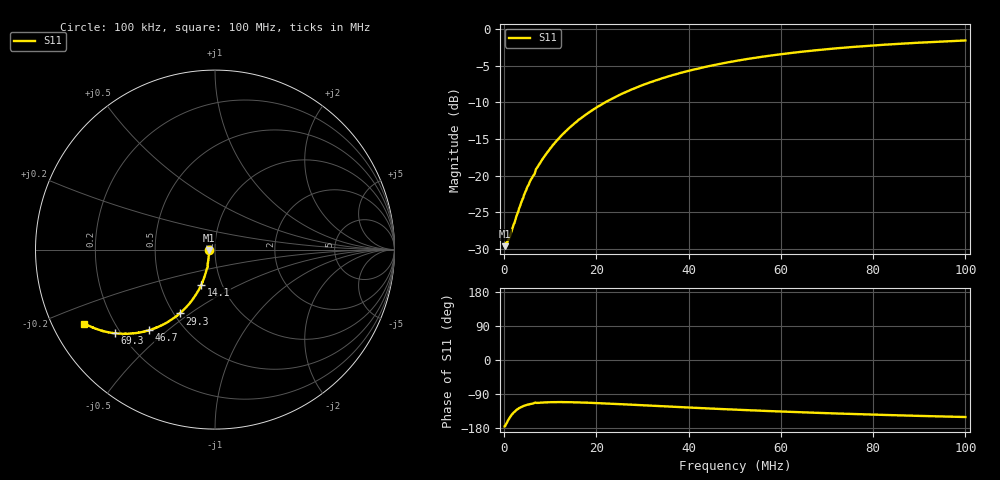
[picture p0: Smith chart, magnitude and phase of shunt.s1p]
# Hz S RI R 50.0
! written by SimSmith version 18.3h
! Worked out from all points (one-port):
!   1000 points, 100 kHz to 100 MHz, reference 50 ohm
!   lowest |S11| = -29.6 dB at 100 kHz (marker M1), VSWR 1.07, Z = 46.8 - j0.253 ohm
!   |S11| at or under -10 dB: start of sweep to 21.87 MHz
!   S11 on the Smith chart (normalised r, x): 100 kHz: 0.94, -0.01; 14.1 MHz: 0.80, -0.33; 29.3 MHz: 0.54, -0.46; 46.7 MHz: 0.32, -0.43; 69.3 MHz: 0.18, -0.35; 100 MHz: 0.10, -0.26
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100000  -0.033 -0.0027
500000  -0.0339 -0.00778
1100000  -0.0341 -0.0163
3300000  -0.0364 -0.0485
4700000  -0.0388 -0.0686
5400000  -0.0403 -0.0783
7200000  -0.0449 -0.1048
8600000  -0.0503 -0.1238
1e7  -0.0557 -0.1428
1.1e7  -0.0605 -0.1567
1.26e7  -0.0687 -0.1775
1.41e7  -0.077 -0.1968
1.61e7  -0.0894 -0.223
1.9e7  -0.1095 -0.2564
2.17e7  -0.1303 -0.2853
2.51e7  -0.1588 -0.3196
2.93e7  -0.1971 -0.3559
3.29e7  -0.2315 -0.3827
3.76e7  -0.2769 -0.4113
4.12e7  -0.3122 -0.4288
4.67e7  -0.3656 -0.4485
5.01e7  -0.397 -0.457
5.56e7  -0.4466 -0.4655
6.26e7  -0.505 -0.4691
6.93e7  -0.5561 -0.4659
7.51e7  -0.5956 -0.4601
8.76e7  -0.6688 -0.439
1e8  -0.7277 -0.4119
